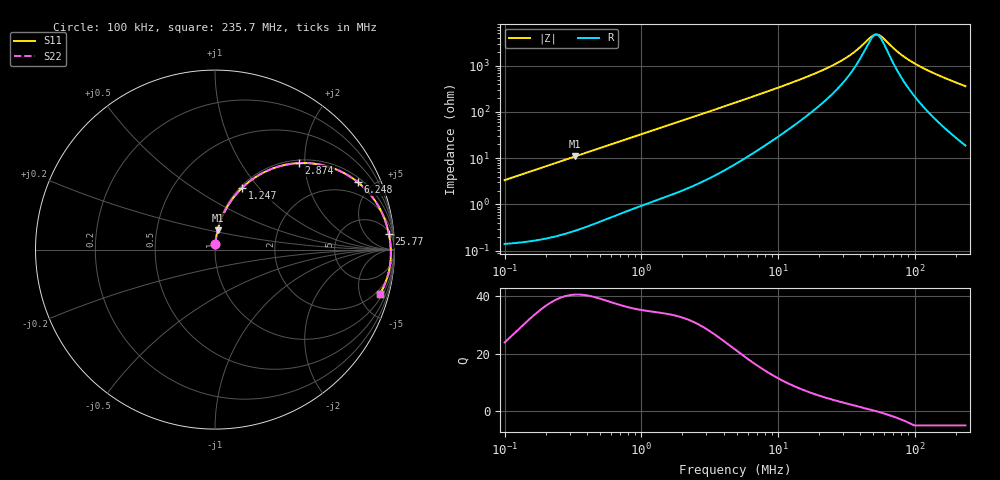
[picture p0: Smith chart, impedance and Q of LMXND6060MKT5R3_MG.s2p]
! LMXND6060MKT5R3_MG  S-PARAMETER MODEL  ( General Type )
! Model Generated by TAIYO YUDEN Corporation (http://www.ty-top.com)
! Version 1.0
! TAIYO YUDEN Control No. 191025NI43SB-FBB
! Copyright(c) 2019 TAIYO YUDEN CO.,LTD. All Rights Reserved.
! Product Description (link to TY-COMPAS)
! https://ds.yuden.co.jp/TYCOMPAS/or/detail?pn=LMXND6060MKT5R3MMG&u=M
! Products Name : Inductors
! Characteristics :
!  Inductance : 5.3 uH , SRF(min) : 34 MHz , DC Resistance(max) : 0.15 Ohm
!  Rated Current : Saturation :1500 mA , Temp Rise : 1550 mA
!  Case Size : 6.0 x 6.0 / 0.236 x 0.236 [mm/inch] , Thickness : 1.2 / 0.047 [mm/inch]
!  (Conditions: Temperature = 25 degC , DC Bias Current/Voltage = 0A / 0V)
! External Node Assignments :
!  1  o---GGG---o  2
! GND o---------o GND
! Frequency Range : 0.1MHz  -  235.669543MHz  [ 402 STEP ]
# MHz S RI R 50
! Freq[MHz].  S11 Real  S11 Imag  S21 Real  S21 Imag  S12 Real  S12 Imag  S22 Real  S22 Imag
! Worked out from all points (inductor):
!   401 points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, 100 kHz to 235.7 MHz, reference 50 ohm
!   read as one part in series: L = 5.33 uH near 104 kHz
!   highest Q = 40.7 at 326.8 kHz (marker M1), where L = 5.31 uH
!   self-resonance near 52.26 MHz
!   S11 on the Smith chart (normalised r, x): 100 kHz: 1.00, +0.07; 1.247 MHz: 1.02, +0.82; 2.874 MHz: 1.06, +1.87; 6.248 MHz: 1.23, +4.10; 25.77 MHz: 6, +20; 235.7 MHz: 1.38, -7.25
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0.1  0.00251 0.0333  0.9975 -0.0333  0.9975 -0.0333  0.00251 0.0333
0.326796  0.0143 0.1072  0.9857 -0.1072  0.9857 -0.1072  0.0143 0.1072
0.367165  0.0176 0.1199  0.9824 -0.1199  0.9824 -0.1199  0.0176 0.1199
0.73853  0.0618 0.2275  0.9382 -0.2275  0.9382 -0.2275  0.0618 0.2275
1.24738  0.1504 0.3433  0.8496 -0.3433  0.8496 -0.3433  0.1504 0.3433
1.348099  0.1703 0.3616  0.8297 -0.3616  0.8297 -0.3616  0.1703 0.3616
1.911945  0.2861 0.437  0.7139 -0.437  0.7139 -0.437  0.2861 0.437
2.874228  0.4684 0.4822  0.5316 -0.4822  0.5316 -0.4822  0.4684 0.4822
4.854581  0.707 0.4325  0.293 -0.4325  0.293 -0.4325  0.707 0.4325
6.248152  0.7949 0.3765  0.2051 -0.3765  0.2051 -0.3765  0.7949 0.3765
9.956113  0.8984 0.2619  0.1016 -0.2619  0.1016 -0.2619  0.8984 0.2619
17.8243  0.9544 0.1432  0.0456 -0.1432  0.0456 -0.1432  0.9544 0.1432
25.7749  0.9689 0.0866  0.0311 -0.0866  0.0311 -0.0866  0.9689 0.0866
35.16326  0.9754 0.0466  0.0246 -0.0466  0.0246 -0.0466  0.9754 0.0466
47.04901  0.9787 0.0122  0.0213 -0.0122  0.0213 -0.0122  0.9787 0.0122
50.84796  0.9792 0.00319  0.0208 -0.00319  0.0208 -0.00319  0.9792 0.00319
56.03086  0.9797 -0.00819  0.0203 0.00819  0.0203 0.00819  0.9797 -0.00819
65.44454  0.9799 -0.0269  0.0201 0.0269  0.0201 0.0269  0.9799 -0.0269
81.02364  0.9789 -0.0541  0.0211 0.0541  0.0211 0.0541  0.9789 -0.0541
106.3267  0.9744 -0.093  0.0256 0.093  0.0256 0.093  0.9744 -0.093
153.7541  0.9593 -0.1565  0.0407 0.1565  0.0407 0.1565  0.9593 -0.1565
235.6695  0.9183 -0.2492  0.0817 0.2492  0.0817 0.2492  0.9183 -0.2492
